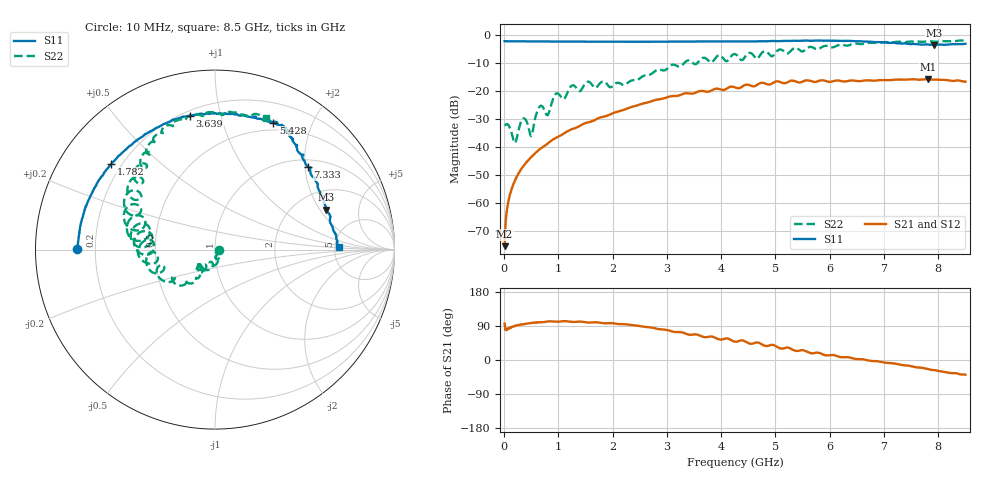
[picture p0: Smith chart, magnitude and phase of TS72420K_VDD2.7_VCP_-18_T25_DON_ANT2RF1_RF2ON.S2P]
!Agilent Technologies,E5071C,MY46417908,A.11.23
!Date: Thu Oct 03 16:40:55 2019
!Data & Calibration Information:
!Freq	S11:SOLT2(ON)	S21:SOLT2(ON)	S12:SOLT2(ON)	S22:SOLT2(ON)
!PortZ  Port1:50+j0  Port2:50+j0
!Above PortZ is port z conversion or system Z0 setting when saving the data.
!When reading, reference impedance value at option line is always used.
# Hz S dB R 50
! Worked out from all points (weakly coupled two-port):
!   1601 points, 10 MHz to 8.5 GHz, reference 50 ohm
!   highest |S21| = -15.82 dB at 7.815 GHz (marker M1); lowest = -75.2 dB at 10 MHz (marker M2)
!   lowest |S11| = -3.6 dB at 7.922 GHz (marker M3), VSWR 4.86, Z = 146 + j115 ohm
!   |S11| at or under -10 dB: nowhere
!   |S22| runs from -38.5 to -2.0 dB; largest |S21 - S12| = 0.0022
!   S11 on the Smith chart (normalised r, x): 10 MHz: 0.13, +0.00; 1.782 GHz: 0.16, +0.35; 3.639 GHz: 0.23, +0.80; 5.428 GHz: 0.41, +1.48; 7.333 GHz: 1.16, +2.07; 8.5 GHz: 5.45, +0.26
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1e7  -2.30 179.9  -75.22 95.8  -74.85 85.1  -32.37 -0.5
1.16125e8  -2.34 177.3  -56.45 84.6  -56.42 85.9  -33.60 -33.4
2.063312e8  -2.35 175.2  -51.59 89.6  -51.61 90.0  -38.46 -18.3
3.389875e8  -2.36 172.1  -47.14 94.1  -47.16 93.9  -30.04 -34.8
4.98175e8  -2.36 168.9  -43.56 97.8  -43.59 97.7  -36.09 -52.4
6.626688e8  -2.39 165.1  -40.63 99.4  -40.66 99.3  -25.43 -67.5
8.006312e8  -2.40 162.1  -38.76 101.6  -38.78 101.4  -28.63 -80.2
9.545125e8  -2.42 158.8  -36.67 101.2  -36.70 101.0  -21.01 -93.3
1.426769e9  -2.48 148.4  -32.08 101.1  -32.08 100.9  -19.51 -117.3
1.782288e9  -2.50 140.3  -29.38 97.8  -29.35 97.6  -17.00 -127.0
2.222706e9  -2.52 130.1  -26.59 94.4  -26.56 94.4  -17.86 -125.9
2.843538e9  -2.48 116.2  -23.03 81.6  -22.97 81.7  -12.42 -129.3
3.639475e9  -2.38 100.7  -19.99 62.5  -19.98 62.7  -8.45 -161.7
4.255e9  -2.39 87.7  -18.72 48.4  -18.71 48.5  -6.90 172.6
4.992569e9  -2.26 73.3  -16.71 37.8  -16.70 38.0  -6.65 166.5
5.427681e9  -2.18 65.3  -16.97 24.2  -16.94 24.3  -5.17 143.3
5.671769e9  -2.16 62.7  -16.62 17.6  -16.62 17.8  -4.41 138.1
7.088538e9  -2.92 48.1  -16.16 -8.1  -16.20 -8.1  -2.70 109.4
7.332625e9  -3.18 41.8  -15.97 -13.4  -15.97 -13.6  -2.52 104.0
7.815494e9  -3.49 25.5  -15.82 -24.1  -15.75 -24.2  -2.31 92.5
7.921619e9  -3.63 19.7  -15.99 -26.5  -15.89 -26.6  -2.45 87.3
8.5e9  -3.21 1.0  -16.70 -38.6  -16.78 -38.5  -2.11 68.7
